//DB987.AWL
// ***************************************************************************


DATA_BLOCK "XC_REBU_SR"
TITLE = Cross Coupling jobs

AUTHOR: 	SIEMENS
FAMILY: 	SISTARS7
NAME:		XCREBUSR
VERSION: 	4.02

//$NOW_HOW_PROTECT

//
// Datum		Name			Aktion
// ----------------------------------------------------------------------------
// 19.05.99 	Mahler		Neu

  STRUCT

        RecvData		: ARRAY[1..15] of "XC_BUFF_SR_UDT" ;

END_STRUCT ;

BEGIN

END_DATA_BLOCK

